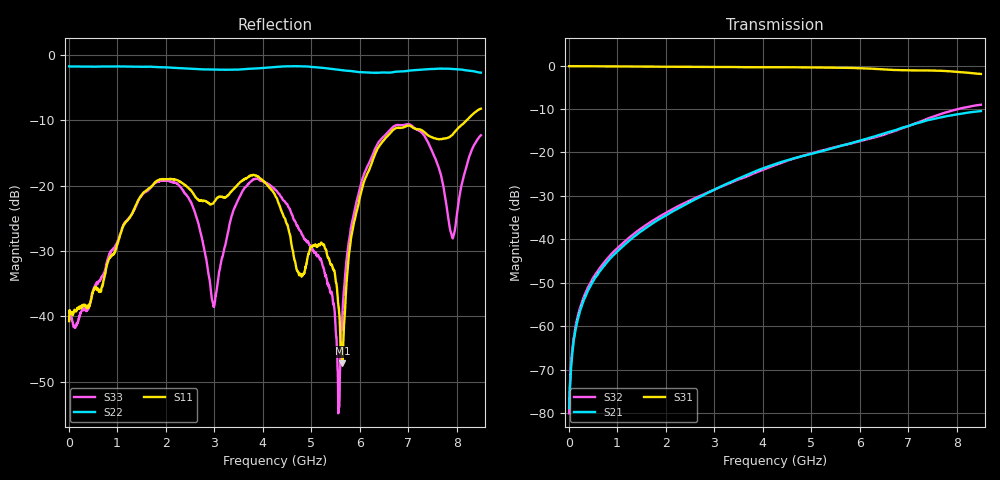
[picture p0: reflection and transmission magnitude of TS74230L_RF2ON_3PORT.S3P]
!Agilent Technologies,E5071C,MY46522130,B.12.04
!Date: Fri Aug 01 10:37:34 2025
!Data & Calibration Information:
!Freq	S11:SOLT3(ON)	S13:SOLT3(ON)	S14:SOLT3(ON)
!	S31:SOLT3(ON)	S33:SOLT3(ON)	S34:SOLT3(ON)
!	S41:SOLT3(ON)	S43:SOLT3(ON)	S44:SOLT3(ON)
!PortZ  Port1:50+j0  Port3:50+j0  Port4:50+j0
!Above PortZ is port z conversion or system Z0 setting when saving the data.
!When reading, reference impedance value at option line is always used.
# Hz S dB R 50
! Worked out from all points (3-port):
!   1601 points, 10 MHz to 8.5 GHz, reference 50 ohm
!   strongest paths, dB at 10 MHz, 2.132 GHz, 4.255 GHz, 6.378 GHz, 8.5 GHz:
!     S31: -0.1, -0.3, -0.4, -0.8, -1.9
!     S21: -78.9, -33.7, -22.7, -16.1, -10.5
!     S32: -80.1, -33.1, -22.9, -16.3, -9.0
!   lowest |S11| = -47.2 dB at 5.645 GHz (marker M1), VSWR 1.01, Z = 49.7 - j0.316 ohm
!   |S11| at or under -10 dB: start of sweep to 8.2 GHz
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1e7  -40.74 22.5  -81.15 34.8  -0.13 -0.4
     -78.87 41.7  -1.70 179.4  -79.18 37.9
     -0.13 -0.4  -80.08 36.9  -40.44 21.3
2.2225e8  -38.53 -19.3  -57.10 89.7  -0.14 -4.5
          -57.18 89.5  -1.73 174.9  -56.24 87.6
          -0.14 -4.5  -56.29 88.2  -39.93 -20.3
8.430812e8  -31.11 -102.4  -44.61 98.5  -0.18 -17.0
            -44.59 98.5  -1.73 161.0  -43.91 93.6
            -0.17 -17.0  -43.90 93.6  -30.41 -81.5
2.2174e9  -19.10 -118.7  -33.14 97.4  -0.28 -44.4
          -33.14 97.4  -1.95 130.5  -32.63 84.1
          -0.28 -44.4  -32.61 84.2  -19.58 -134.3
2.992112e9  -22.57 -67.1  -28.64 90.9  -0.30 -60.3
            -28.64 91.0  -2.20 109.7  -28.65 74.4
            -0.30 -60.3  -28.64 74.3  -38.47 131.5
4.255e9  -21.42 -11.8  -22.70 69.2  -0.37 -87.1
         -22.69 69.0  -1.80 72.6  -22.96 53.2
         -0.38 -87.1  -22.92 53.4  -20.59 29.7
5.645238e9  -47.20 -133.3  -18.44 40.7  -0.50 -119.6
            -18.39 40.9  -2.30 40.8  -18.36 22.1
            -0.50 -119.6  -18.37 21.7  -39.69 -30.0
6.382806e9  -14.14 -54.4  -16.05 25.4  -0.80 -138.7
            -16.05 25.7  -2.69 14.3  -16.39 8.4
            -0.80 -138.7  -16.30 7.9  -13.41 -60.6
7.916312e9  -12.18 5.7  -11.33 -21.9  -1.36 178.3
            -11.41 -22.2  -2.10 -20.8  -10.27 -34.6
            -1.36 178.3  -10.32 -35.0  -28.01 -16.1
8.5e9  -8.19 33.6  -10.54 -42.8  -1.92 158.2
       -10.47 -43.2  -2.67 -29.0  -9.05 -59.5
       -1.92 158.1  -9.01 -59.4  -12.27 53.4
